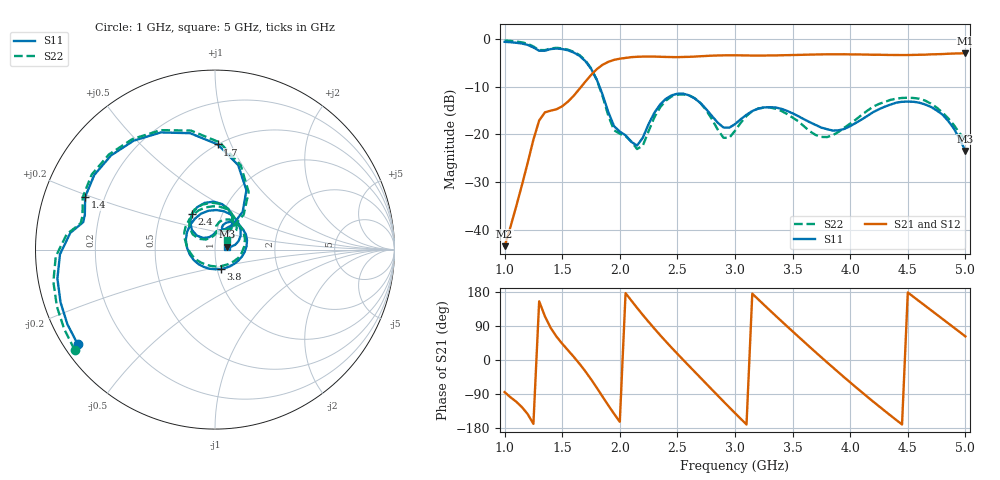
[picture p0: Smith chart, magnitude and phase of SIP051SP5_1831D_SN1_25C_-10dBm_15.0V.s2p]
# GHz  S  dB  R  50
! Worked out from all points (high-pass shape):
!   81 points, 1 GHz to 5 GHz, reference 50 ohm
!   highest |S21| = -3.02 dB at 5 GHz (marker M1); lowest = -43.4 dB at 1 GHz (marker M2)
!   |S21| within 3 dB of the highest: 1.819 GHz to end of sweep
!   lowest |S11| = -23.4 dB at 5 GHz (marker M3), VSWR 1.14, Z = 57 + j1.87 ohm
!   |S11| at or under -10 dB: 1.824 GHz to end of sweep
!   |S22| runs from -23.1 to -0.3 dB; largest |S21 - S12| = 0.0021
!   S11 on the Smith chart (normalised r, x): 1 GHz: 0.04, -0.31; 1.4 GHz: 0.13, +0.19; 1.7 GHz: 0.50, +0.89; 2.4 GHz: 0.72, +0.30; 3.8 GHz: 1.04, -0.23; 5 GHz: 1.14, +0.04
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1  -0.64 -145.4  -43.36 -84.7  -43.27 -88.7  -0.35 -144.5
1.3  -2.50 168.3  -17.08 154.9  -17.10 154.8  -2.35 168.9
1.4  -2.15 157.9  -15.03 84.8  -15.04 84.9  -2.02 158.3
1.55  -2.41 126.8  -13.13 25.9  -13.12 26.0  -2.28 126.8
1.7  -4.64 88.5  -8.99 -29.5  -8.98 -29.4  -4.47 87.5
1.85  -11.64 53.9  -5.43 -96.5  -5.43 -96.5  -11.97 50.6
2.05  -20.18 87.1  -4.00 176.5  -4.00 176.5  -20.32 86.3
2.2  -20.68 135.7  -3.72 118.8  -3.71 118.9  -22.34 132.4
2.35  -13.73 132.2  -3.76 65.7  -3.75 65.7  -14.33 138.3
2.4  -12.55 123.1  -3.79 48.9  -3.80 48.8  -12.93 128.3
2.55  -11.47 91.4  -3.80 0.5  -3.81 0.5  -11.63 94.4
2.75  -14.71 57.0  -3.59 -62.4  -3.58 -62.4  -14.90 55.8
3  -17.85 72.7  -3.45 -140.1  -3.44 -140.0  -19.24 87.3
3.2  -14.61 54.0  -3.50 160.5  -3.51 160.6  -14.60 64.1
3.4  -14.62 16.3  -3.44 103.5  -3.44 103.5  -15.05 19.1
3.7  -18.01 -47.4  -3.28 20.5  -3.29 20.6  -20.11 -68.3
3.8  -18.90 -73.9  -3.25 -6.5  -3.25 -6.5  -20.55 -104.4
4.1  -16.86 -169.6  -3.28 -84.7  -3.28 -84.8  -15.90 171.7
4.35  -13.76 123.0  -3.38 -146.4  -3.39 -146.4  -12.77 121.7
4.65  -13.73 56.5  -3.32 143.4  -3.31 143.5  -12.92 67.3
4.85  -17.16 19.5  -3.13 97.1  -3.14 97.2  -16.61 39.1
5  -23.43 14.1  -3.02 62.2  -3.03 62.4  -21.18 39.6
